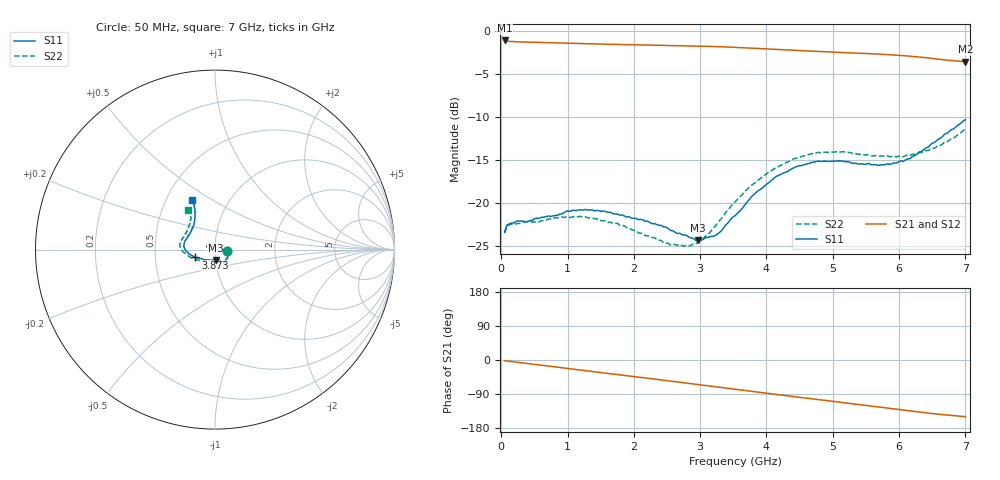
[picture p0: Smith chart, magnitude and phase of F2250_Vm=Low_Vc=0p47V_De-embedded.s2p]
! Integrated Device Technology
! Corporate Headquarters
! 6024 Silver Creek Valley Road
! San Jose, CA 95138  USA
! Phone:  1-408-284-8200
! Toll Free:  1-800-223-1366
! Webpage:  http://www.idt.com/
! Timing and RF Division
! 515 Groton Road, Suite 102
! Westford, MA 01886-6024
! Device:  F2250
! Description: Voltage Variable RF Attenuator
! Frequency:  50.0 -  6000.00 MHz
! Package:  3x3 mm Thin QFN Plastic Package: 16 pin
! Ports:  2 RF, 3 DC
!  Pin  1  = GND
!  Pin  2  = NC
!  Pin  3  = RF1  = Port 1
!  Pin  4  = NC
!  Pin  5  = GND
!  Pin  6  = GND
!  Pin  7  = GND
!  Pin  8  = GND
!  Pin  9  = NC
!  Pin 10  = RF2  = Port 2
!  Pin 11  = NC
!  Pin 12  = GND
!  Pin 13  = GND
!  Pin 14  = VCNTRL
!  Pin 15  = VDD
!  Pin 16  = VMODE
! Vcntrl:  0.470 Volts
! Vmode:  +0.000 Volts
! Vdd:  +3.30  Volts
! Current:  1.130 mA
! Data:  The device was measured on a the F2250 evaluation board which has
!  individual transmission lines to the RF pins.  Data was collected
!  using a calibrated network analyzer.  The evaluation board was
!  de-embedded using a TRL calibration technique.
!  The reference plane is the edge of the package pin.
! Misc:  SN 10
!  Action Tracker AT0258
! Date Measured:  2014-11-26
! Date:  2015-10-15  MJV
! Note:
!  Integrated Device Technology supplies this data as a sample of measured
!  data at the package pin for this product.  Your particular data for this
!  product may vary.
!  Data was taken at 25 degrees C.
!  Integrated Device Technology reserves the right to change this data at anytime.
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# GHz S dB R 50
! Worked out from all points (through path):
!   201 points, 50 MHz to 7 GHz, reference 50 ohm
!   highest |S21| = -1.05 dB at 50 MHz (marker M1); lowest = -3.5 dB at 7 GHz (marker M2)
!   group delay of S21, straight-line fit = 60.1 ps
!   lowest |S11| = -24.4 dB at 2.969 GHz (marker M3), VSWR 1.13, Z = 50 - j6.04 ohm
!   |S11| at or under -10 dB: start of sweep to end of sweep
!   |S22| runs from -25.1 to -11.4 dB; largest |S21 - S12| = 0.0004
!   S11 on the Smith chart (normalised r, x): 50 MHz: 1.14, -0.02; 3.873 GHz: 0.80, -0.07; 7 GHz: 0.67, +0.41
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0.05  -23.38 -8.1  -1.05 -1.8  -1.04 -1.8  -23.56 -8.9
0.08475  -22.60 -8.1  -1.12 -2.5  -1.12 -2.5  -22.72 -8.3
0.15425  -22.37 -10.2  -1.17 -4.0  -1.17 -4.0  -22.48 -10.1
0.71025  -21.53 -34.0  -1.30 -16.2  -1.30 -16.2  -21.87 -36.1
1.2315  -20.85 -50.7  -1.42 -27.4  -1.42 -27.4  -21.67 -56.6
1.75275  -21.33 -57.5  -1.51 -38.5  -1.51 -38.5  -22.39 -64.9
2.37825  -22.61 -59.0  -1.60 -51.8  -1.60 -51.8  -24.36 -69.9
2.552  -23.22 -62.7  -1.62 -55.6  -1.62 -55.6  -24.93 -75.7
2.7605  -23.77 -71.6  -1.66 -60.2  -1.66 -60.2  -25.07 -87.3
2.969  -24.40 -86.4  -1.70 -64.8  -1.70 -64.8  -24.57 -103.5
3.247  -23.73 -114.3  -1.76 -71.0  -1.76 -71.0  -22.54 -126.7
3.525  -21.51 -139.5  -1.85 -77.2  -1.85 -77.2  -19.91 -143.8
3.8725  -18.60 -158.2  -1.98 -84.8  -1.98 -84.8  -17.37 -159.6
4.1505  -16.90 -169.0  -2.09 -90.9  -2.09 -90.9  -15.87 -169.7
4.4285  -15.87 -177.0  -2.20 -96.9  -2.20 -96.9  -14.82 -177.1
4.7065  -15.27 176.0  -2.30 -103.0  -2.30 -103.0  -14.28 176.7
5.15825  -15.14 165.1  -2.46 -112.7  -2.46 -112.7  -14.04 167.3
5.85325  -15.51 141.6  -2.71 -127.6  -2.71 -127.6  -14.62 151.9
6.166  -14.82 130.2  -2.88 -134.4  -2.88 -134.4  -14.46 142.9
6.444  -13.49 121.4  -3.09 -140.2  -3.09 -140.2  -13.89 133.5
6.82625  -11.36 115.3  -3.41 -146.9  -3.40 -146.9  -12.44 125.5
7  -10.30 114.5  -3.53 -149.5  -3.53 -149.5  -11.42 124.0
